(* Logix 5000 AddOnInstructionDefinition export; software revision 16.04 *)

ADD_ON_INSTRUCTION AMCI_ANG1E_Program_Assembled_Move   (* revision 1.0 *)
VAR_INPUT
   Axis_Status_Bits : INT; {required}
   slot_axis_number : INT; {required}
   Number_of_Segments : DINT; {required}
   Segment_1_Distance : DINT; {required}
   Segment_1_Programmed_Speed : DINT; {required}
   Segment_1_Acceleration : INT; {required}
   Segment_1_Deceleration : INT; {required}
   Segment_2_Distance : DINT; {required}
   Segment_2_Programmed_Speed : DINT; {required}
   Segment_2_Acceleration : INT; {required}
   Segment_2_Deceleration : INT; {required}
   Segment_3_Distance : DINT; {required}
   Segment_3_Programmed_Speed : DINT; {required}
   Segment_3_Acceleration : INT; {required}
   Segment_3_Deceleration : INT; {required}
   Segment_4_Distance : DINT; {required}
   Segment_4_Programmed_Speed : DINT; {required}
   Segment_4_Acceleration : INT; {required}
   Segment_4_Deceleration : INT; {required}
   Segment_5_Distance : DINT; {required}
   Segment_5_Programmed_Speed : DINT; {required}
   Segment_5_Acceleration : INT; {required}
   Segment_5_Deceleration : INT; {required}
   Segment_6_Distance : DINT; {required}
   Segment_6_Programmed_Speed : DINT; {required}
   Segment_6_Acceleration : INT; {required}
   Segment_6_Deceleration : INT; {required}
   Segment_7_Distance : DINT; {required}
   Segment_7_Programmed_Speed : DINT; {required}
   Segment_7_Acceleration : INT; {required}
   Segment_7_Deceleration : INT; {required}
   Segment_8_Distance : DINT; {required}
   Segment_8_Programmed_Speed : DINT; {required}
   Segment_8_Acceleration : INT; {required}
   Segment_8_Deceleration : INT; {required}
   Segment_9_Distance : DINT; {required}
   Segment_9_Programmed_Speed : DINT; {required}
   Segment_9_Acceleration : INT; {required}
   Segment_9_Deceleration : INT; {required}
   Segment_10_Distance : DINT; {required}
   Segment_10_Programmed_Speed : DINT; {required}
   Segment_10_Acceleration : INT; {required}
   Segment_10_Deceleration : INT; {required}
   Segment_11_Distance : DINT; {required}
   Segment_11_Programmed_Speed : DINT; {required}
   Segment_11_Acceleration : INT; {required}
   Segment_11_Deceleration : INT; {required}
   Segment_12_Distance : DINT; {required}
   Segment_12_Programmed_Speed : DINT; {required}
   Segment_12_Acceleration : INT; {required}
   Segment_12_Deceleration : INT; {required}
   Segment_13_Distance : DINT; {required}
   Segment_13_Programmed_Speed : DINT; {required}
   Segment_13_Acceleration : INT; {required}
   Segment_13_Deceleration : INT; {required}
   Segment_14_Distance : DINT; {required}
   Segment_14_Programmed_Speed : DINT; {required}
   Segment_14_Acceleration : INT; {required}
   Segment_14_Deceleration : INT; {required}
   Segment_15_Distance : DINT; {required}
   Segment_15_Programmed_Speed : DINT; {required}
   Segment_15_Acceleration : INT; {required}
   Segment_15_Deceleration : INT; {required}
   Segment_16_Distance : DINT; {required}
   Segment_16_Programmed_Speed : DINT; {required}
   Segment_16_Acceleration : INT; {required}
   Segment_16_Deceleration : INT; {required}
END_VAR
VAR_IN_OUT
   AMCI_ANG1E_output_data : INT[10]; {required}
END_VAR
VAR_OUTPUT
   Assembled_Move_Programmed : BOOL; {visible}
END_VAR
VAR
   command_data_block : INT[10];
   Assembled_Move_setup : INT[10];
   Assembled_Move_counter : COUNTER;
   Programmed_Speed : DINT;
   Distance : DINT;
   upper_result_X_1000 : DINT;
   index : DINT;
END_VAR

ROUTINE Logic   (* ladder *)
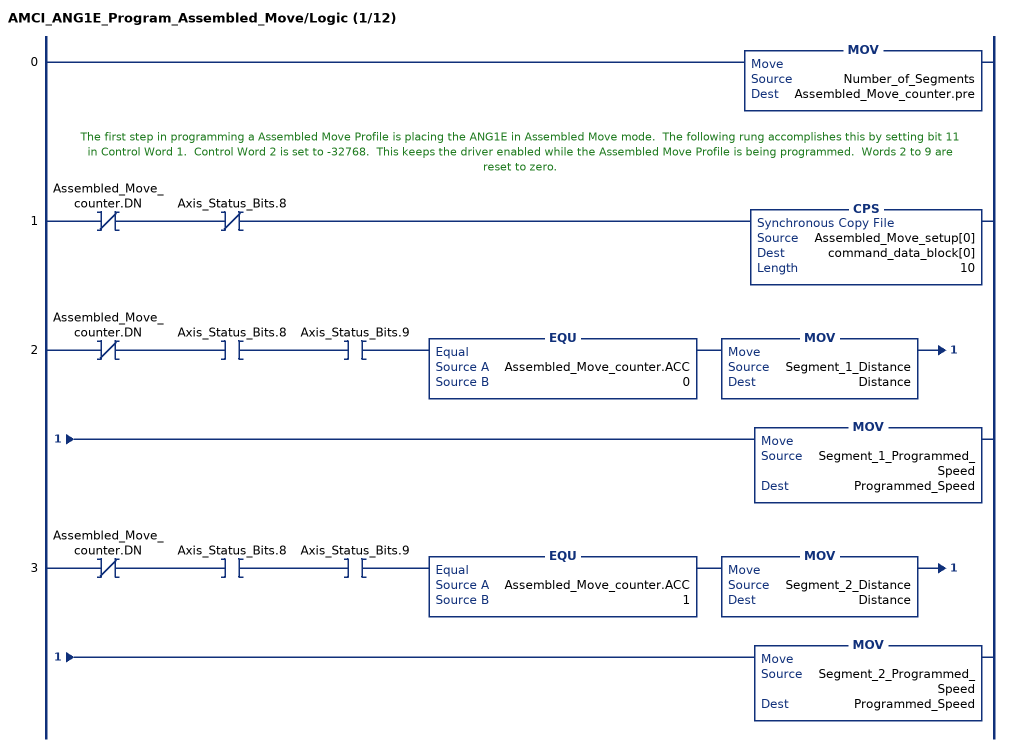
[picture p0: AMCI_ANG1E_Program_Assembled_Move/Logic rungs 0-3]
   0: MOV(Number_of_Segments,Assembled_Move_counter.pre);
   // The first step in programming a Assembled Move Profile is placing the ANG1E in Assembled Move mode.  The following rung accomplishes this by setting bit 11 in Control Word 1.  Control Word 2 is set to -32768.  This keeps the driver enabled while the Assembled Move Profile is being programmed.  Words 2 to 9 are reset to zero.
   1: XIO(Assembled_Move_counter.DN)XIO(Axis_Status_Bits.8)CPS(Assembled_Move_setup[0],command_data_block[0],10);
   2: XIO(Assembled_Move_counter.DN)XIC(Axis_Status_Bits.8)XIC(Axis_Status_Bits.9)EQU(Assembled_Move_counter.ACC,0)MOV(Segment_1_Distance,Distance)MOV(Segment_1_Programmed_Speed,Programmed_Speed);
   3: XIO(Assembled_Move_counter.DN)XIC(Axis_Status_Bits.8)XIC(Axis_Status_Bits.9)EQU(Assembled_Move_counter.ACC,1)MOV(Segment_2_Distance,Distance)MOV(Segment_2_Programmed_Speed,Programmed_Speed);
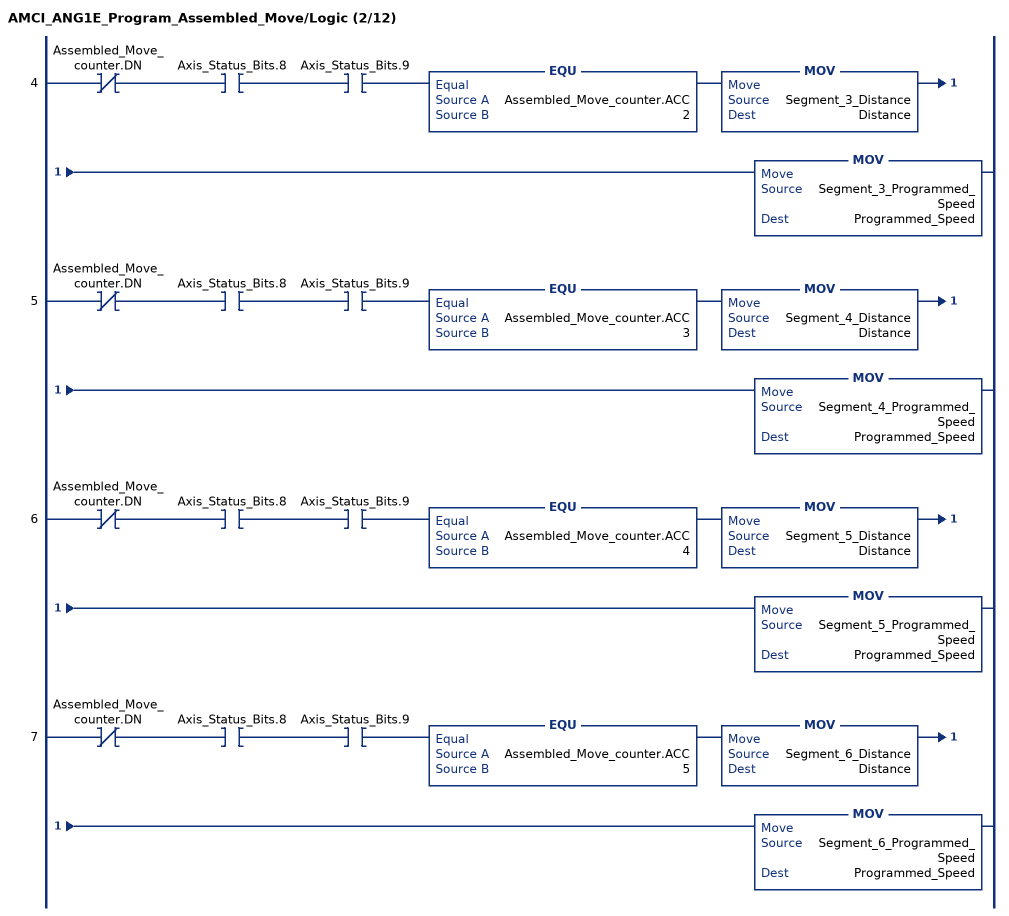
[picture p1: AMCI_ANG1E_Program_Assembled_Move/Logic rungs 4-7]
   4: XIO(Assembled_Move_counter.DN)XIC(Axis_Status_Bits.8)XIC(Axis_Status_Bits.9)EQU(Assembled_Move_counter.ACC,2)MOV(Segment_3_Distance,Distance)MOV(Segment_3_Programmed_Speed,Programmed_Speed);
   5: XIO(Assembled_Move_counter.DN)XIC(Axis_Status_Bits.8)XIC(Axis_Status_Bits.9)EQU(Assembled_Move_counter.ACC,3)MOV(Segment_4_Distance,Distance)MOV(Segment_4_Programmed_Speed,Programmed_Speed);
   6: XIO(Assembled_Move_counter.DN)XIC(Axis_Status_Bits.8)XIC(Axis_Status_Bits.9)EQU(Assembled_Move_counter.ACC,4)MOV(Segment_5_Distance,Distance)MOV(Segment_5_Programmed_Speed,Programmed_Speed);
   7: XIO(Assembled_Move_counter.DN)XIC(Axis_Status_Bits.8)XIC(Axis_Status_Bits.9)EQU(Assembled_Move_counter.ACC,5)MOV(Segment_6_Distance,Distance)MOV(Segment_6_Programmed_Speed,Programmed_Speed);
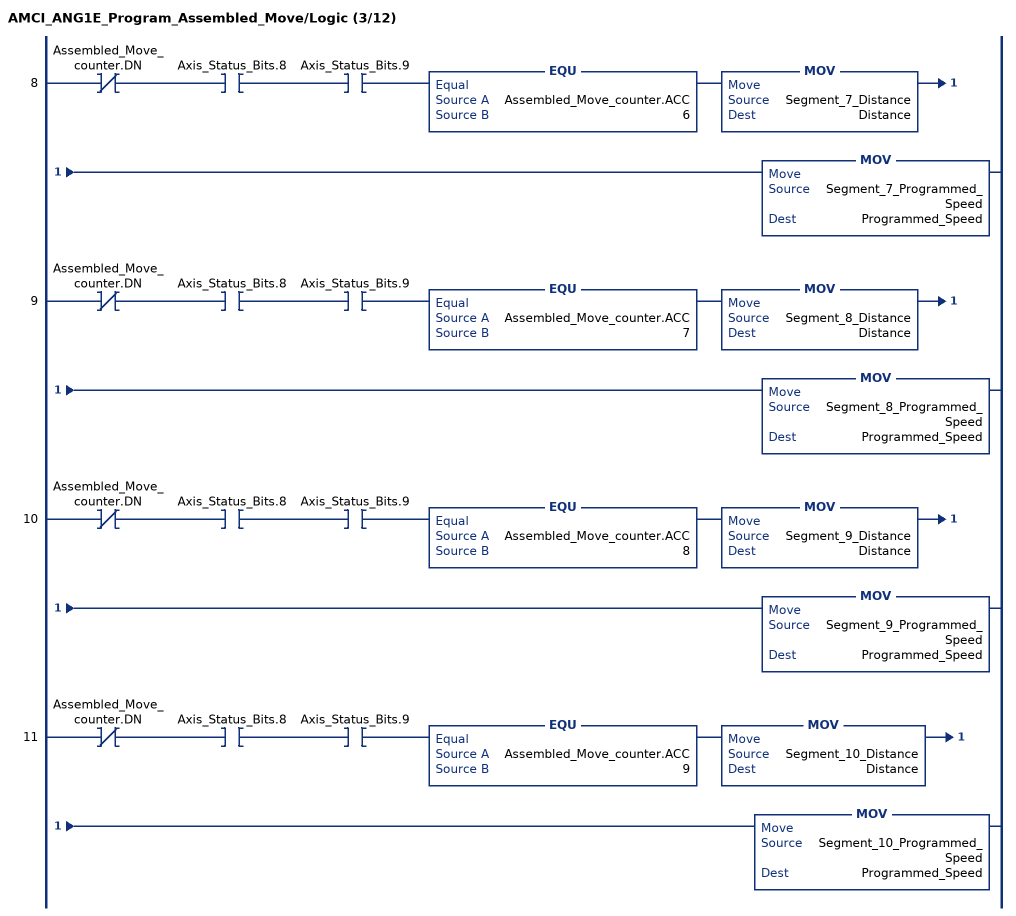
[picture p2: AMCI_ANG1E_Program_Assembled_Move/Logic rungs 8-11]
   8: XIO(Assembled_Move_counter.DN)XIC(Axis_Status_Bits.8)XIC(Axis_Status_Bits.9)EQU(Assembled_Move_counter.ACC,6)MOV(Segment_7_Distance,Distance)MOV(Segment_7_Programmed_Speed,Programmed_Speed);
   9: XIO(Assembled_Move_counter.DN)XIC(Axis_Status_Bits.8)XIC(Axis_Status_Bits.9)EQU(Assembled_Move_counter.ACC,7)MOV(Segment_8_Distance,Distance)MOV(Segment_8_Programmed_Speed,Programmed_Speed);
   10: XIO(Assembled_Move_counter.DN)XIC(Axis_Status_Bits.8)XIC(Axis_Status_Bits.9)EQU(Assembled_Move_counter.ACC,8)MOV(Segment_9_Distance,Distance)MOV(Segment_9_Programmed_Speed,Programmed_Speed);
   11: XIO(Assembled_Move_counter.DN)XIC(Axis_Status_Bits.8)XIC(Axis_Status_Bits.9)EQU(Assembled_Move_counter.ACC,9)MOV(Segment_10_Distance,Distance)MOV(Segment_10_Programmed_Speed,Programmed_Speed);
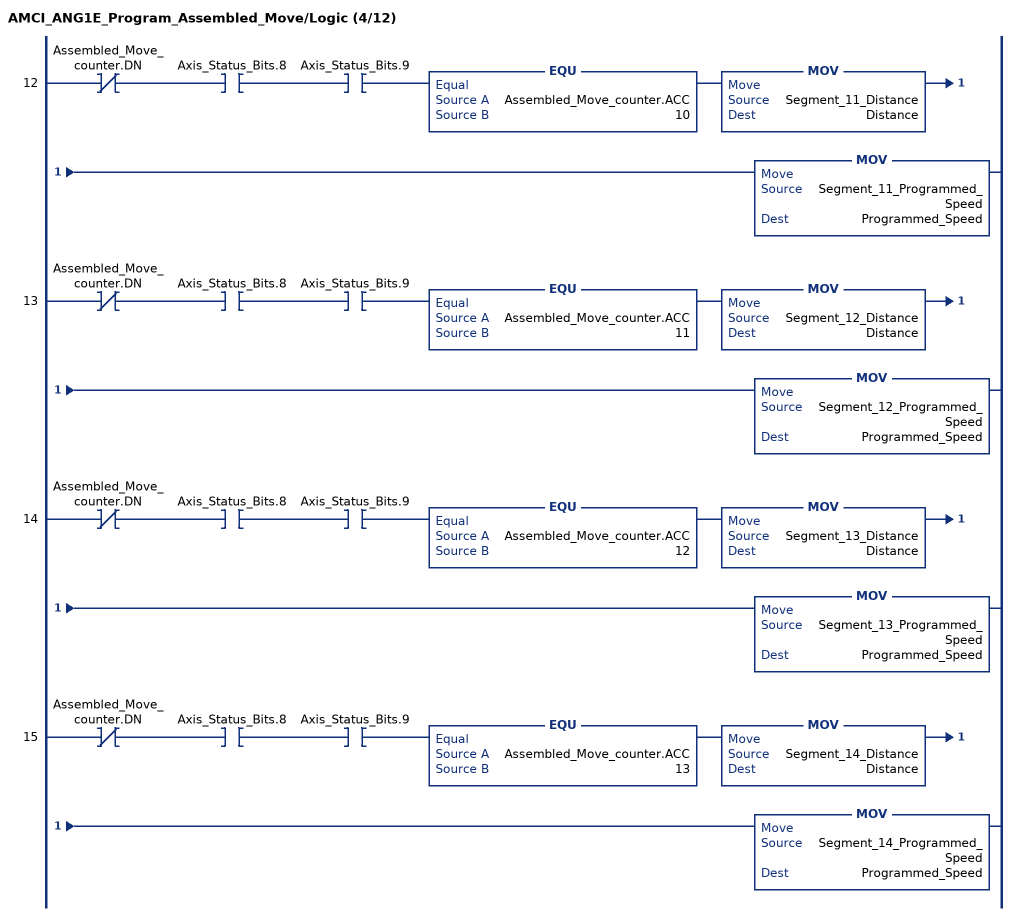
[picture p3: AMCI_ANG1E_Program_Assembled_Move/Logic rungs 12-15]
   12: XIO(Assembled_Move_counter.DN)XIC(Axis_Status_Bits.8)XIC(Axis_Status_Bits.9)EQU(Assembled_Move_counter.ACC,10)MOV(Segment_11_Distance,Distance)MOV(Segment_11_Programmed_Speed,Programmed_Speed);
   13: XIO(Assembled_Move_counter.DN)XIC(Axis_Status_Bits.8)XIC(Axis_Status_Bits.9)EQU(Assembled_Move_counter.ACC,11)MOV(Segment_12_Distance,Distance)MOV(Segment_12_Programmed_Speed,Programmed_Speed);
   14: XIO(Assembled_Move_counter.DN)XIC(Axis_Status_Bits.8)XIC(Axis_Status_Bits.9)EQU(Assembled_Move_counter.ACC,12)MOV(Segment_13_Distance,Distance)MOV(Segment_13_Programmed_Speed,Programmed_Speed);
   15: XIO(Assembled_Move_counter.DN)XIC(Axis_Status_Bits.8)XIC(Axis_Status_Bits.9)EQU(Assembled_Move_counter.ACC,13)MOV(Segment_14_Distance,Distance)MOV(Segment_14_Programmed_Speed,Programmed_Speed);
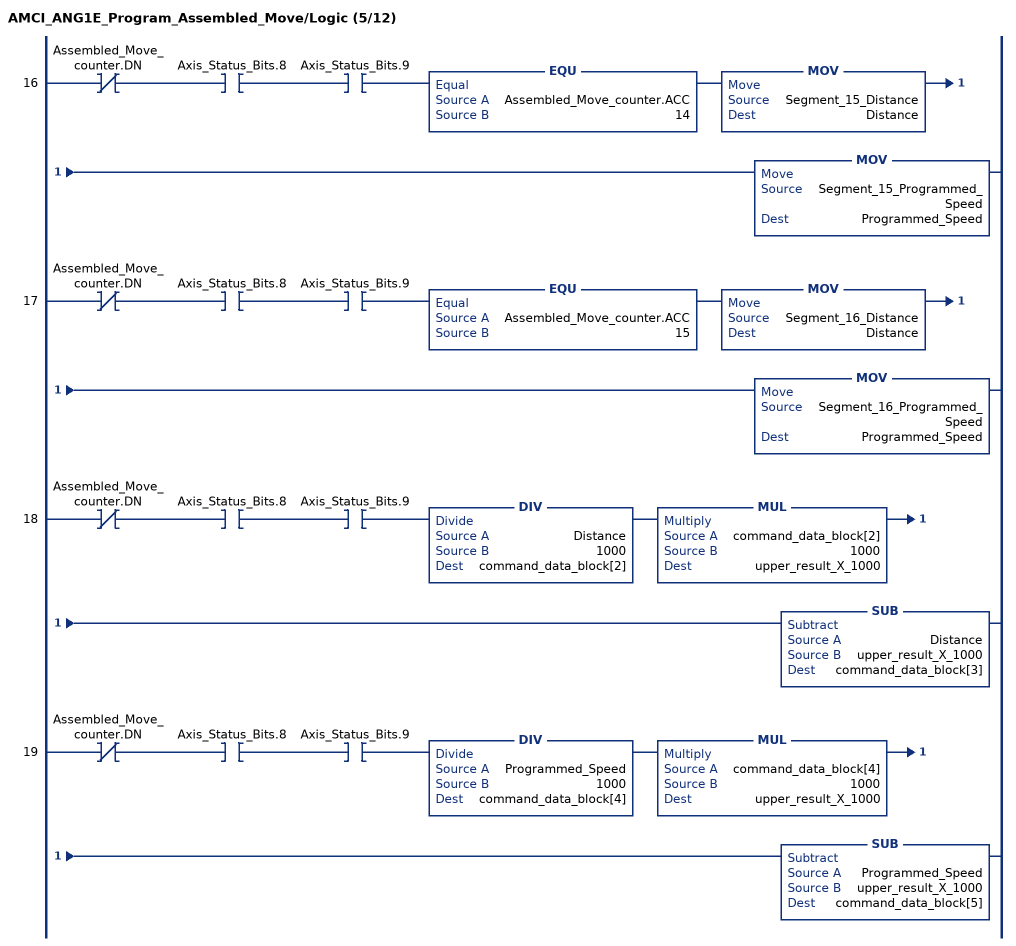
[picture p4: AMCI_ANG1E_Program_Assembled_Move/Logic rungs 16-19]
   16: XIO(Assembled_Move_counter.DN)XIC(Axis_Status_Bits.8)XIC(Axis_Status_Bits.9)EQU(Assembled_Move_counter.ACC,14)MOV(Segment_15_Distance,Distance)MOV(Segment_15_Programmed_Speed,Programmed_Speed);
   17: XIO(Assembled_Move_counter.DN)XIC(Axis_Status_Bits.8)XIC(Axis_Status_Bits.9)EQU(Assembled_Move_counter.ACC,15)MOV(Segment_16_Distance,Distance)MOV(Segment_16_Programmed_Speed,Programmed_Speed);
   18: XIO(Assembled_Move_counter.DN)XIC(Axis_Status_Bits.8)XIC(Axis_Status_Bits.9)DIV(Distance,1000,command_data_block[2])MUL(command_data_block[2],1000,upper_result_X_1000)SUB(Distance,upper_result_X_1000,command_data_block[3]);
   19: XIO(Assembled_Move_counter.DN)XIC(Axis_Status_Bits.8)XIC(Axis_Status_Bits.9)DIV(Programmed_Speed,1000,command_data_block[4])MUL(command_data_block[4],1000,upper_result_X_1000)SUB(Programmed_Speed,upper_result_X_1000,command_data_block[5]);
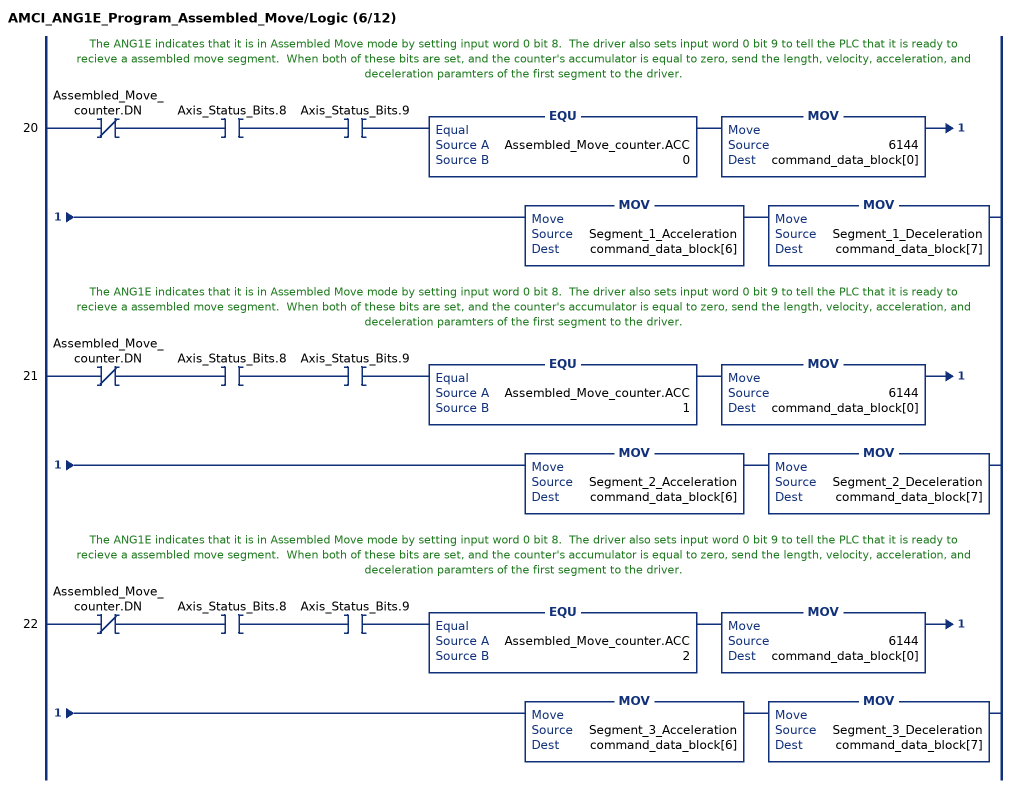
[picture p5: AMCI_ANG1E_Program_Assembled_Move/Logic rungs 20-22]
   // The ANG1E indicates that it is in Assembled Move mode by setting input word 0 bit 8.  The driver also sets input word 0 bit 9 to tell the PLC that it is ready to recieve a assembled move segment.  When both of these bits are set, and the counter's accumulator is equal to zero, send the length, velocity, acceleration, and deceleration paramters of the first segment to the driver.
   20: XIO(Assembled_Move_counter.DN)XIC(Axis_Status_Bits.8)XIC(Axis_Status_Bits.9)EQU(Assembled_Move_counter.ACC,0)MOV(6144,command_data_block[0])MOV(Segment_1_Acceleration,command_data_block[6])MOV(Segment_1_Deceleration,command_data_block[7]);
   // The ANG1E indicates that it is in Assembled Move mode by setting input word 0 bit 8.  The driver also sets input word 0 bit 9 to tell the PLC that it is ready to recieve a assembled move segment.  When both of these bits are set, and the counter's accumulator is equal to zero, send the length, velocity, acceleration, and deceleration paramters of the first segment to the driver.
   21: XIO(Assembled_Move_counter.DN)XIC(Axis_Status_Bits.8)XIC(Axis_Status_Bits.9)EQU(Assembled_Move_counter.ACC,1)MOV(6144,command_data_block[0])MOV(Segment_2_Acceleration,command_data_block[6])MOV(Segment_2_Deceleration,command_data_block[7]);
   // The ANG1E indicates that it is in Assembled Move mode by setting input word 0 bit 8.  The driver also sets input word 0 bit 9 to tell the PLC that it is ready to recieve a assembled move segment.  When both of these bits are set, and the counter's accumulator is equal to zero, send the length, velocity, acceleration, and deceleration paramters of the first segment to the driver.
   22: XIO(Assembled_Move_counter.DN)XIC(Axis_Status_Bits.8)XIC(Axis_Status_Bits.9)EQU(Assembled_Move_counter.ACC,2)MOV(6144,command_data_block[0])MOV(Segment_3_Acceleration,command_data_block[6])MOV(Segment_3_Deceleration,command_data_block[7]);
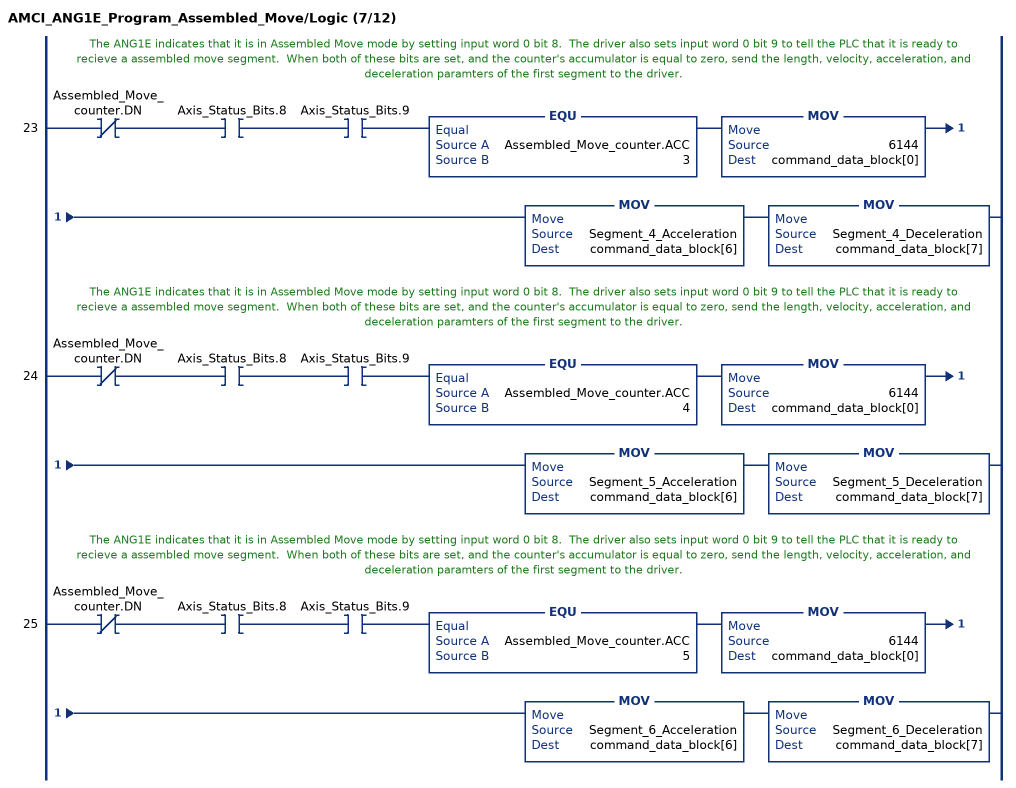
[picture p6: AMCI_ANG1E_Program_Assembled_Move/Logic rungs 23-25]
   // The ANG1E indicates that it is in Assembled Move mode by setting input word 0 bit 8.  The driver also sets input word 0 bit 9 to tell the PLC that it is ready to recieve a assembled move segment.  When both of these bits are set, and the counter's accumulator is equal to zero, send the length, velocity, acceleration, and deceleration paramters of the first segment to the driver.
   23: XIO(Assembled_Move_counter.DN)XIC(Axis_Status_Bits.8)XIC(Axis_Status_Bits.9)EQU(Assembled_Move_counter.ACC,3)MOV(6144,command_data_block[0])MOV(Segment_4_Acceleration,command_data_block[6])MOV(Segment_4_Deceleration,command_data_block[7]);
   // The ANG1E indicates that it is in Assembled Move mode by setting input word 0 bit 8.  The driver also sets input word 0 bit 9 to tell the PLC that it is ready to recieve a assembled move segment.  When both of these bits are set, and the counter's accumulator is equal to zero, send the length, velocity, acceleration, and deceleration paramters of the first segment to the driver.
   24: XIO(Assembled_Move_counter.DN)XIC(Axis_Status_Bits.8)XIC(Axis_Status_Bits.9)EQU(Assembled_Move_counter.ACC,4)MOV(6144,command_data_block[0])MOV(Segment_5_Acceleration,command_data_block[6])MOV(Segment_5_Deceleration,command_data_block[7]);
   // The ANG1E indicates that it is in Assembled Move mode by setting input word 0 bit 8.  The driver also sets input word 0 bit 9 to tell the PLC that it is ready to recieve a assembled move segment.  When both of these bits are set, and the counter's accumulator is equal to zero, send the length, velocity, acceleration, and deceleration paramters of the first segment to the driver.
   25: XIO(Assembled_Move_counter.DN)XIC(Axis_Status_Bits.8)XIC(Axis_Status_Bits.9)EQU(Assembled_Move_counter.ACC,5)MOV(6144,command_data_block[0])MOV(Segment_6_Acceleration,command_data_block[6])MOV(Segment_6_Deceleration,command_data_block[7]);
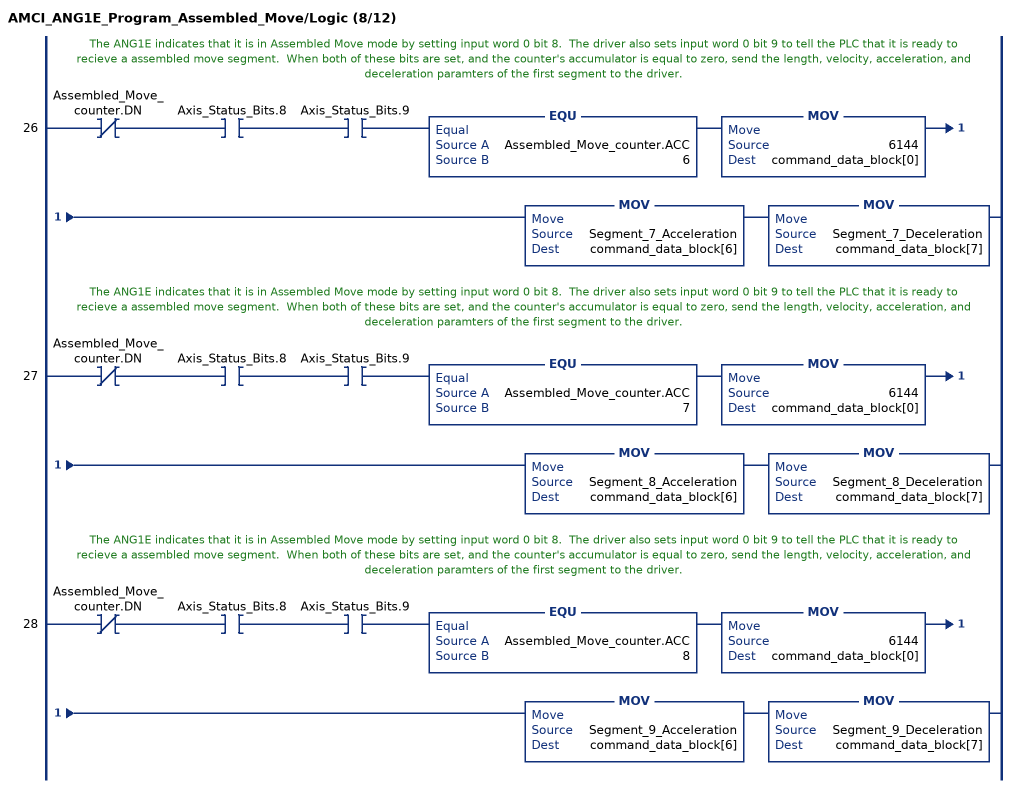
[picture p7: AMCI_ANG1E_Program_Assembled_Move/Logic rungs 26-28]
   // The ANG1E indicates that it is in Assembled Move mode by setting input word 0 bit 8.  The driver also sets input word 0 bit 9 to tell the PLC that it is ready to recieve a assembled move segment.  When both of these bits are set, and the counter's accumulator is equal to zero, send the length, velocity, acceleration, and deceleration paramters of the first segment to the driver.
   26: XIO(Assembled_Move_counter.DN)XIC(Axis_Status_Bits.8)XIC(Axis_Status_Bits.9)EQU(Assembled_Move_counter.ACC,6)MOV(6144,command_data_block[0])MOV(Segment_7_Acceleration,command_data_block[6])MOV(Segment_7_Deceleration,command_data_block[7]);
   // The ANG1E indicates that it is in Assembled Move mode by setting input word 0 bit 8.  The driver also sets input word 0 bit 9 to tell the PLC that it is ready to recieve a assembled move segment.  When both of these bits are set, and the counter's accumulator is equal to zero, send the length, velocity, acceleration, and deceleration paramters of the first segment to the driver.
   27: XIO(Assembled_Move_counter.DN)XIC(Axis_Status_Bits.8)XIC(Axis_Status_Bits.9)EQU(Assembled_Move_counter.ACC,7)MOV(6144,command_data_block[0])MOV(Segment_8_Acceleration,command_data_block[6])MOV(Segment_8_Deceleration,command_data_block[7]);
   // The ANG1E indicates that it is in Assembled Move mode by setting input word 0 bit 8.  The driver also sets input word 0 bit 9 to tell the PLC that it is ready to recieve a assembled move segment.  When both of these bits are set, and the counter's accumulator is equal to zero, send the length, velocity, acceleration, and deceleration paramters of the first segment to the driver.
   28: XIO(Assembled_Move_counter.DN)XIC(Axis_Status_Bits.8)XIC(Axis_Status_Bits.9)EQU(Assembled_Move_counter.ACC,8)MOV(6144,command_data_block[0])MOV(Segment_9_Acceleration,command_data_block[6])MOV(Segment_9_Deceleration,command_data_block[7]);
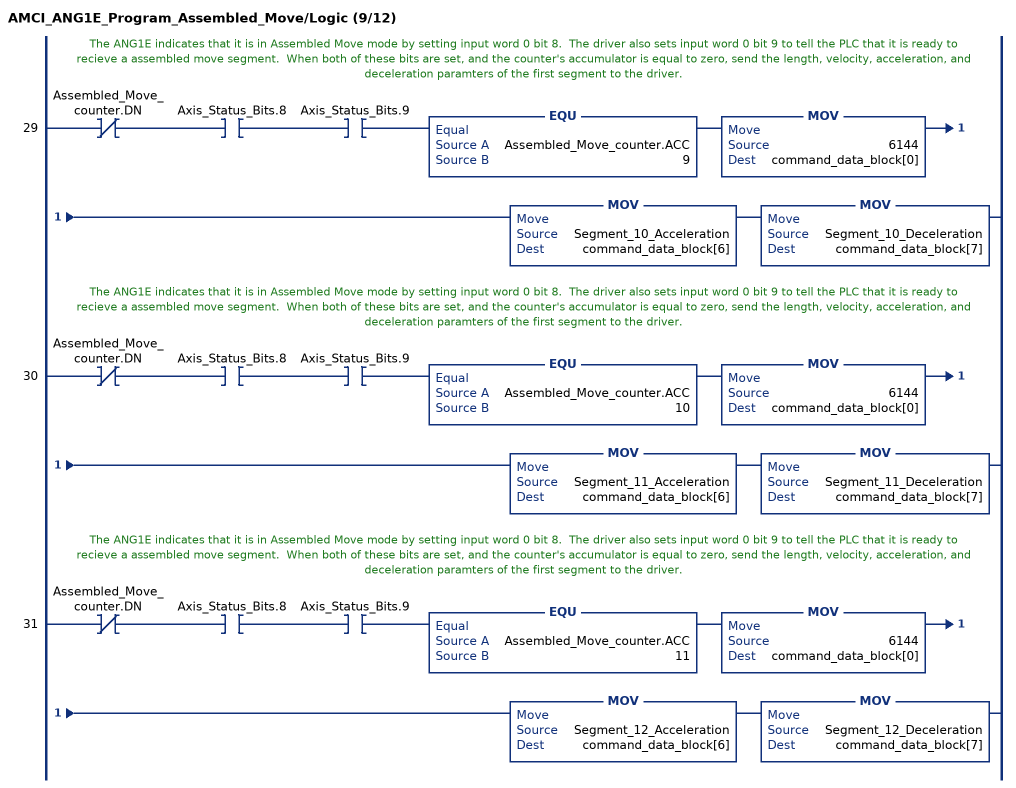
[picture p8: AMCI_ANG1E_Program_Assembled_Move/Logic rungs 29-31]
   // The ANG1E indicates that it is in Assembled Move mode by setting input word 0 bit 8.  The driver also sets input word 0 bit 9 to tell the PLC that it is ready to recieve a assembled move segment.  When both of these bits are set, and the counter's accumulator is equal to zero, send the length, velocity, acceleration, and deceleration paramters of the first segment to the driver.
   29: XIO(Assembled_Move_counter.DN)XIC(Axis_Status_Bits.8)XIC(Axis_Status_Bits.9)EQU(Assembled_Move_counter.ACC,9)MOV(6144,command_data_block[0])MOV(Segment_10_Acceleration,command_data_block[6])MOV(Segment_10_Deceleration,command_data_block[7]);
   // The ANG1E indicates that it is in Assembled Move mode by setting input word 0 bit 8.  The driver also sets input word 0 bit 9 to tell the PLC that it is ready to recieve a assembled move segment.  When both of these bits are set, and the counter's accumulator is equal to zero, send the length, velocity, acceleration, and deceleration paramters of the first segment to the driver.
   30: XIO(Assembled_Move_counter.DN)XIC(Axis_Status_Bits.8)XIC(Axis_Status_Bits.9)EQU(Assembled_Move_counter.ACC,10)MOV(6144,command_data_block[0])MOV(Segment_11_Acceleration,command_data_block[6])MOV(Segment_11_Deceleration,command_data_block[7]);
   // The ANG1E indicates that it is in Assembled Move mode by setting input word 0 bit 8.  The driver also sets input word 0 bit 9 to tell the PLC that it is ready to recieve a assembled move segment.  When both of these bits are set, and the counter's accumulator is equal to zero, send the length, velocity, acceleration, and deceleration paramters of the first segment to the driver.
   31: XIO(Assembled_Move_counter.DN)XIC(Axis_Status_Bits.8)XIC(Axis_Status_Bits.9)EQU(Assembled_Move_counter.ACC,11)MOV(6144,command_data_block[0])MOV(Segment_12_Acceleration,command_data_block[6])MOV(Segment_12_Deceleration,command_data_block[7]);
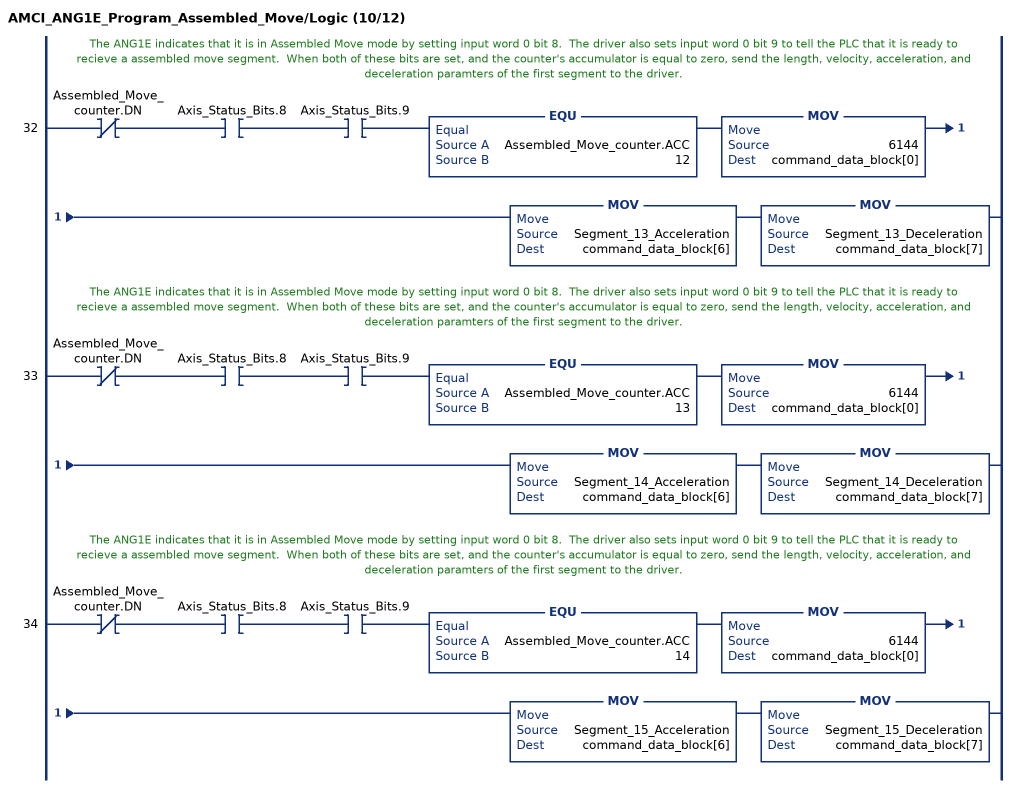
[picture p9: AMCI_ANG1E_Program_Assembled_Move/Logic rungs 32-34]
   // The ANG1E indicates that it is in Assembled Move mode by setting input word 0 bit 8.  The driver also sets input word 0 bit 9 to tell the PLC that it is ready to recieve a assembled move segment.  When both of these bits are set, and the counter's accumulator is equal to zero, send the length, velocity, acceleration, and deceleration paramters of the first segment to the driver.
   32: XIO(Assembled_Move_counter.DN)XIC(Axis_Status_Bits.8)XIC(Axis_Status_Bits.9)EQU(Assembled_Move_counter.ACC,12)MOV(6144,command_data_block[0])MOV(Segment_13_Acceleration,command_data_block[6])MOV(Segment_13_Deceleration,command_data_block[7]);
   // The ANG1E indicates that it is in Assembled Move mode by setting input word 0 bit 8.  The driver also sets input word 0 bit 9 to tell the PLC that it is ready to recieve a assembled move segment.  When both of these bits are set, and the counter's accumulator is equal to zero, send the length, velocity, acceleration, and deceleration paramters of the first segment to the driver.
   33: XIO(Assembled_Move_counter.DN)XIC(Axis_Status_Bits.8)XIC(Axis_Status_Bits.9)EQU(Assembled_Move_counter.ACC,13)MOV(6144,command_data_block[0])MOV(Segment_14_Acceleration,command_data_block[6])MOV(Segment_14_Deceleration,command_data_block[7]);
   // The ANG1E indicates that it is in Assembled Move mode by setting input word 0 bit 8.  The driver also sets input word 0 bit 9 to tell the PLC that it is ready to recieve a assembled move segment.  When both of these bits are set, and the counter's accumulator is equal to zero, send the length, velocity, acceleration, and deceleration paramters of the first segment to the driver.
   34: XIO(Assembled_Move_counter.DN)XIC(Axis_Status_Bits.8)XIC(Axis_Status_Bits.9)EQU(Assembled_Move_counter.ACC,14)MOV(6144,command_data_block[0])MOV(Segment_15_Acceleration,command_data_block[6])MOV(Segment_15_Deceleration,command_data_block[7]);
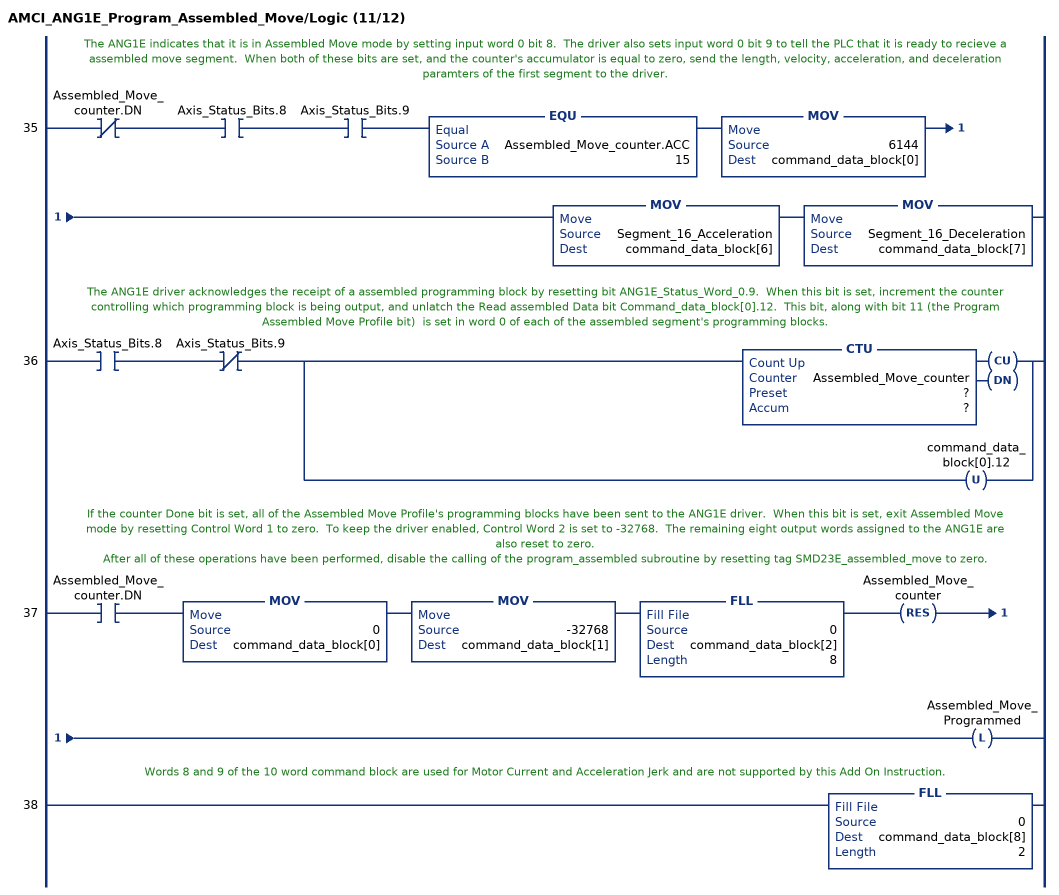
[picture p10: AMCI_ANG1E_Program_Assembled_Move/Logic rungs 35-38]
   // The ANG1E indicates that it is in Assembled Move mode by setting input word 0 bit 8.  The driver also sets input word 0 bit 9 to tell the PLC that it is ready to recieve a assembled move segment.  When both of these bits are set, and the counter's accumulator is equal to zero, send the length, velocity, acceleration, and deceleration paramters of the first segment to the driver.
   35: XIO(Assembled_Move_counter.DN)XIC(Axis_Status_Bits.8)XIC(Axis_Status_Bits.9)EQU(Assembled_Move_counter.ACC,15)MOV(6144,command_data_block[0])MOV(Segment_16_Acceleration,command_data_block[6])MOV(Segment_16_Deceleration,command_data_block[7]);
   // The ANG1E driver acknowledges the receipt of a assembled programming block by resetting bit ANG1E_Status_Word_0.9.  When this bit is set, increment the counter controlling which programming block is being output, and unlatch the Read assembled Data bit Command_data_block[0].12.  This bit, along with bit 11 (the Program Assembled Move Profile bit)  is set in word 0 of each of the assembled segment's programming blocks.
   36: XIC(Axis_Status_Bits.8)XIO(Axis_Status_Bits.9)[CTU(Assembled_Move_counter,?,?) ,OTU(command_data_block[0].12) ];
   // If the counter Done bit is set, all of the Assembled Move Profile's programming blocks have been sent to the ANG1E driver.  When this bit is set, exit Assembled Move mode by resetting Control Word 1 to zero.  To keep the driver enabled, Control Word 2 is set to -32768.  The remaining eight output words assigned to the ANG1E are also reset to zero.
   // After all of these operations have been performed, disable the calling of the program_assembled subroutine by resetting tag SMD23E_assembled_move to zero.
   37: XIC(Assembled_Move_counter.DN)MOV(0,command_data_block[0])MOV(-32768,command_data_block[1])FLL(0,command_data_block[2],8)RES(Assembled_Move_counter)OTL(Assembled_Move_Programmed);
   // Words 8 and 9 of the 10 word command block are used for Motor Current and Acceleration Jerk and are not supported by this Add On Instruction.
   38: FLL(0,command_data_block[8],2);
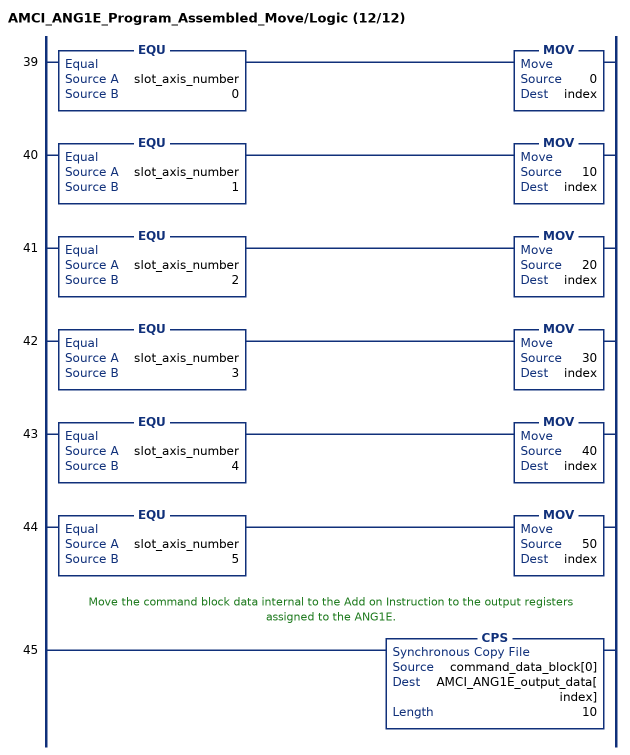
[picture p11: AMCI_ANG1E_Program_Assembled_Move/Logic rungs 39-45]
   39: EQU(slot_axis_number,0)MOV(0,index);
   40: EQU(slot_axis_number,1)MOV(10,index);
   41: EQU(slot_axis_number,2)MOV(20,index);
   42: EQU(slot_axis_number,3)MOV(30,index);
   43: EQU(slot_axis_number,4)MOV(40,index);
   44: EQU(slot_axis_number,5)MOV(50,index);
   // Move the command block data internal to the Add on Instruction to the output registers assigned to the ANG1E.
   45: CPS(command_data_block[0],AMCI_ANG1E_output_data[index],10);
END_ROUTINE
END_ADD_ON_INSTRUCTION
